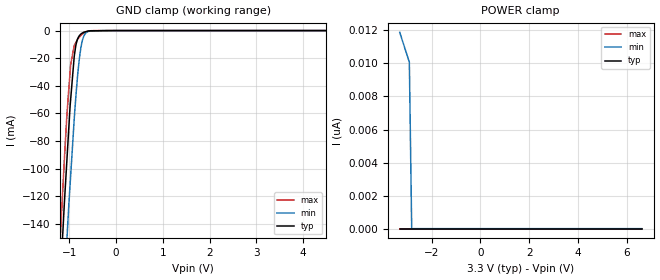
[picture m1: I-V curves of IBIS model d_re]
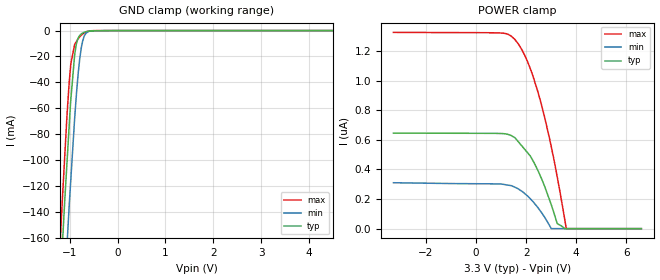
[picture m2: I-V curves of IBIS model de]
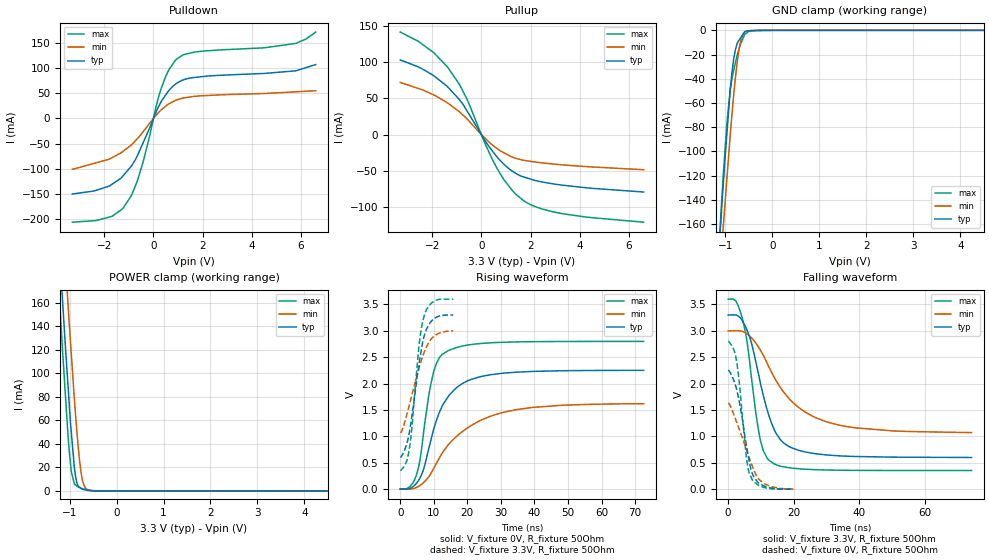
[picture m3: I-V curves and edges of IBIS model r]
|Texas Instruments Incorporated
| Robust Compact 3.3V-supply RS-485
| Marketing part#   Digital Voltage Range   Package-type   #pins
| SN65HVD75D   3V-3.6V   SOIC   8
[IBIS Ver]   3.2
[File name]   sn65hvd75.ibs
|SIMDE Ver   V3.0 - 201101 - RHL4 - Build 457
[File Rev]   1.2
[Date]   3/29/2012
[Source]
| Texas Instruments Incorporated.
| Analog-eLab Design Center, HPA
| 12500 TI Blvd
| Dallas, TX -75243
| e-mail: elab_scm_ibis@list.ti.com
[Notes]   Revision History:
| Rev 1.2: 3/29/2012
| - The VT Tables in the IBIS file are generated with
|   vfixture = Vcm(1.956-TYP, 1.731-SLOW, 2.134-FAST).
| Rev 1.1: 3/27/2012
| - IBIS file is generated with Rload = 27 Ohms &
|   Common Mode Voltage(Vcm) values calculated using the
|   setup from the datasheet.
| Rev 1.0: 3/21/2012
| - Initial version of the model
| - Model generated from simulations in TISPICE
| - Model matched to SPICE simulation
| - C_comp although listed in numerical order of value are
|   obtained from varying PVT conditions. For PVT conditions for
|   each specific value refer the buffer description under
|   respective [Model]. IBIS model user is responsible for using
|   appropriate C_comp to simulate for Signal Integrity.
|* EXCEPTION:   *
|* - For model d_re, there is leakage current in the GND   *
|*   clamp I-V Table because of the pullup on pad.   *
|* - For model de, there is leakage current in the POWER   *
|*   clamp I-V Table because of the pulldown on pad.   *
|* - For models a_b_p and a_b_n, there is leakage current in the   *
|*   POWER clamp I-V Table because of the pulldown resistors and   *
|*   the resistor network connected to pad and in the GND clamp I-V *
|*   table because of the resistor network connected to pad.   *
|* - For a_b_p and a_b_n models, pullup non-montonicity reflects   *
|*   true buffer behavior.   *
[Disclaimer]
| This model is designed as an aid for customers of Texas Instruments.
| TI and its licensors and suppliers make no warranties, either expressed
| or implied, with respect to this  model, including the warranties of
| merchantability or fitness for a particular purpose. The model is
| provided solely on an "as is" basis. The entire risk as to its quality
| and performance is with the customer.
[Copyright]
(C) Copyright 2011 Texas Instruments Incorporated.All rights reserved.
|   SN65HVD75D
[Component]   SN65HVD75D
[Manufacturer]   TI
[Package]   |8 SOIC   -  D package
|   typ   min   max
R_pkg   0.05962   0.05594   0.06721
L_pkg   2.46828nH   2.21379nH   2.98434nH
C_pkg   0.38513pF   0.35622pF   0.44246pF
[Pin]  signal_name   model_name   R_pin   L_pin   C_pin
1   R   r   0.06721   2.98434nH  0.44246pF
2   _RE   d_re   0.05732   2.24625nH  0.35866pF
3   DE   de   0.05594   2.21379nH  0.35622pF
4   D   d_re   0.06108   2.82596nH  0.43337pF
5   GND   gnd   0.02940   2.20778nH  0.47000pF
6   A   a_b_p   0.05797   2.26926nH  0.35995pF
7   B   a_b_n   0.05821   2.27008nH  0.36013pF
8   VCC   power   0.03012   2.24722nH  0.47300pF
[Diff_pin]   inv_pin   vdiff   tdelay_typ   tdelay_min   tdelay_max
6   7   0.2V   NA   NA   NA
| Models and submodels in the file (5): d_re (Input), de (Input), r (3-state), a_b_p (I/O), a_b_n (I/O)
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|   d_re Model
[Model]   d_re
Model_type   Input
Vinl = 0.8
Vinh = 2
|   typ   min   max
|   (nom PVT)   (fast PVT)   (slow PVT)
C_comp   7.616e-13   7.309e-13   8.232e-13
| Where nom  PVT is Nominal Process, 3.3V, 27C
|   Fast PVT is Strong Process,  3.6V, -40C
|   Slow PVT is Weak Process,   3V, 125C
[Voltage Range]   3.3   3   3.6
|Ambient Temperature   25   125   -40
|Junction Temperature
[Temperature Range]   27   125   -40
[Power Clamp Reference]   3.3   3   3.6
[GND Clamp Reference]   0   0   0
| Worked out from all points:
|   GND clamp passes 1 mA (typ) near -0.67 V on its own axis
[GND Clamp]
|   Voltage   I(typ)   I(min)   I(max)
-3.3V     -1.705A    -1.7A      -1.738A
-1.195V   -180.4mA   -237.2mA   -148.9mA
-1.158V   -156.2mA   -213.2mA   -124.7mA
-1.112V   -126.4mA   -185.5mA   -94.94mA
-1.055V   -93.52mA   -150.9mA   -60.84mA
-975.6mV  -50.1mA    -105.4mA   -24.74mA
-897.6mV  -18.42mA   -63.54mA   -10.82mA
-858mV    -9.846mA   -45.32mA   -8.298mA
-792mV    -3.842mA   -21.25mA   -4.834mA
-693mV    -1.196mA   -3.902mA   -1.803mA
-285mV    -93.15uA   -1.769uA   -4.655uA
6.6V      0A         0A         0A
[POWER Clamp]
|   Voltage   I(typ)   I(min)   I(max)
-3.3V     0A         11.88nA    0A
-3.298V   0A         11.87nA    0A
-3V       0A         10.5nA     0A
-2.907V   0A         10.07nA    0A
-2.811V   0A         0A         0A
6.6V      0A         0A         0A
|   de Model
[Model]   de
Model_type   Input
Vinl = 0.8
Vinh = 2
|   typ   min   max
|   (nom PVT)   (fast PVT)   (slow PVT)
C_comp   7.616e-13   7.309e-13   8.232e-13
| Where nom  PVT is Nominal Process, 3.3V, 27C
|   Fast PVT is Strong Process,  3.6V, -40C
|   Slow PVT is Weak Process,   3V, 125C
[Voltage Range]   3.3   3   3.6
|Ambient Temperature   25   125   -40
|Junction Temperature
[Temperature Range]   27   125   -40
[Power Clamp Reference]   3.3   3   3.6
[GND Clamp Reference]   0   0   0
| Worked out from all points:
|   GND clamp passes 1 mA (typ) near -0.67 V on its own axis
[GND Clamp]
|   Voltage   I(typ)   I(min)   I(max)
-3.3V     -1.872A    -1.872A    -1.901A
-1.192V   -192.8mA   -257.5mA   -157.9mA
-1.152V   -164.4mA   -228.9mA   -129.2mA
-1.105V   -132.4mA   -198mA     -97.99mA
-1.055V   -100.7mA   -164.3mA   -64.15mA
-975.6mV  -52.85mA   -114.1mA   -25.21mA
-897.6mV  -18.95mA   -68.11mA   -10.83mA
-858mV    -9.962mA   -48.2mA    -8.3mA
-792mV    -3.844mA   -22.19mA   -4.834mA
-693mV    -1.196mA   -3.944mA   -1.803mA
-285mV    -92.82uA   -1.603uA   -3.947uA
6.6V      0A         0A         0A
[POWER Clamp]
|   Voltage   I(typ)   I(min)   I(max)
-3.3V     645nA      310.1nA    1.325uA
939.6mV   642.6nA    301.8nA    1.322uA
1.422V    626.9nA    289.4nA    1.298uA
1.685V    587.5nA    268.5nA    1.248uA
1.948V    534.5nA    236.2nA    1.169uA
2.168V    490.1nA    201.3nA    1.079uA
2.473V    391.4nA    141.5nA    921.2nA
2.736V    286.6nA    77.39nA    753.7nA
3.003V    161.7nA    0A         553nA
3.241V    34.27nA    0A         349.4nA
3.604V    0A         0A         0A
6.6V      0A         0A         0A
|   r Model
[Model]   r
Model_type   3-state
Polarity   Non-Inverting
Vmeas = 1.65
Vref = 1.65
Cref = 2pF
Rref = 50
|   typ   min   max
|   (nom PVT)   (fast PVT)   (slow PVT)
C_comp   2.780e-12   2.415e-12   2.953e-12
|ON state : BUFFER OUTPUT TURNED HIGH
|C_comp   2.780e-12   2.415e-12   2.953e-12
|OFF state: BUFFER IN HIGH IMPEDANCE
|C_comp   2.507e-12   2.233e-12   2.622e-12
| Where nom  PVT is Nominal Process, 3.3V, 27C
|   Fast PVT is Strong Process,  3.6V, -40C
|   Slow PVT is Weak Process,   3V, 125C
[Voltage Range]   3.3   3   3.6
|Ambient Temperature   25   125   -40
|Junction Temperature
[Temperature Range]   27   125   -40
[Pullup Reference]   3.3   3   3.6
[Pulldown Reference]   0   0   0
[Power Clamp Reference]   3.3   3   3.6
[GND Clamp Reference]   0   0   0
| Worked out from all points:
|   slope of the pulldown table from 0 to 0.495 V, typ, clamps not added: 10.7 ohm
|   slope of the pullup table from 0 to 0.495 V, typ, clamps not added: 20.1 ohm
|   GND clamp passes 1 mA (typ) near -0.58 V on its own axis
|   POWER clamp passes 1 mA (typ) near -0.68 V on its own axis
|   falling waveform, V_fixture 3.3V, R_fixture 50Ohm: 20-80 % time 6.84ns typ, 13.6ns min, 4.27ns max; typ from 3.3 V to 0.6 V
|   rising waveform, V_fixture 0V, R_fixture 50Ohm: 20-80 % time 7.58ns typ, 14.3ns min, 4.13ns max; typ from 0 V to 2.25 V
|   rising waveform, V_fixture 3.3V, R_fixture 50Ohm: 20-80 % time 3.71ns typ, 5.13ns min, 2.82ns max; typ from 0.601 V to 3.3 V
|   falling waveform, V_fixture 0V, R_fixture 50Ohm: 20-80 % time 3.74ns typ, 5.69ns min, 2.65ns max; typ from 2.25 V to 0 V
[Pulldown]
|   Voltage   I(typ)   I(min)   I(max)
-3.3V     -149.9mA   -101.1mA   -205.7mA
-1.685V   -130.5mA   -77.82mA   -194mA
-1.249V   -114.5mA   -65.67mA   -178.9mA
-896.4mV  -94.5mA    -52.63mA   -153mA
-673.2mV  -76.17mA   -41.18mA   -126.5mA
-428.4mV  -49.17mA   -26.94mA   -87.39mA
306mV     32.4mA     16.57mA    58.12mA
633.6mV   55.83mA    28.96mA    96.76mA
939.6mV   69.38mA    36.44mA    117.2mA
1.706V    81.24mA    43.83mA    131.5mA
5.771V    94.09mA    52.55mA    148.3mA
6.6V      106.6mA    54.73mA    170.9mA
[GND Clamp]
|   Voltage   I(typ)   I(min)   I(max)
-3.3V     -1.695A    -1.623A    -1.774A
-1.168V   -200.9mA   -231.6mA   -200.3mA
-1.069V   -140.8mA   -175.9mA   -134.8mA
-1.044V   -126.3mA   -161.7mA   -119.2mA
-968.4mV  -85.6mA    -123mA     -76.83mA
-896.4mV  -49.17mA   -86.21mA   -48.82mA
-825mV    -24.16mA   -54.22mA   -33.37mA
-714mV    -8.511mA   -16.89mA   -15.83mA
-645mV    -4.403mA   -5.377mA   -8.386mA
-590.7mV  -1.17mA    -1.748mA   -3.672mA
-439.2mV  -342.9uA   -399uA     -96.91uA
6.6V      0A         0A         0A
[Pullup]
|   Voltage   I(typ)   I(min)   I(max)
-3.3V     103.4mA    72.24mA    141.8mA
-2.56V    93.6mA     63.82mA    129mA
-1.926V   81.19mA    54.79mA    113mA
-1.375V   66.16mA    43.89mA    93.4mA
-896.4mV  48.62mA    31.69mA    69.68mA
-572.4mV  32.23mA    21.44mA    48.14mA
172.8mV   -9.472mA   -5.689mA   -14.19mA
633.6mV   -30.76mA   -19.2mA    -46.34mA
1.246V    -50.27mA   -30.87mA   -76.8mA
1.706V    -58.35mA   -35.31mA   -91.08mA
3.287V    -69.84mA   -41.73mA   -109.2mA
6.6V      -79.34mA   -48.49mA   -121mA
[POWER Clamp]
|   Voltage   I(typ)   I(min)   I(max)
-3.3V     1.726A     1.768A     1.712A
-1.277V   248.4mA    321.2mA    207.4mA
-1.155V   166.1mA    237.6mA    123.2mA
-1.037V   92.04mA    161.7mA    49.65mA
-964.8mV  50.85mA    117.8mA    16.73mA
-897.6mV  19.75mA    78.19mA    5.955mA
-867.9mV  11.2mA     62.54mA    4.838mA
-816mV    4.299mA    37.54mA    3.5mA
-745.8mV  1.73mA     13.5mA     2.285mA
-657mV    822.1uA    2.18mA     1.302mA
-486mV    181.5uA    98.8uA     38.01uA
6.6V      0A         0A         0A
[Ramp]
R_load = 50
|   typ   min   max
dV/dt_r   1.35124/7.57455e-09   0.974782/1.44691e-08   1.67977/4.13078e-09
dV/dt_f   1.6192/6.82107e-09   1.15786/1.36049e-08   1.9482/4.2637e-09
[Falling Waveform]
V_fixture = 3.3V
V_fixture_min = 3V
V_fixture_max = 3.6V
R_fixture = 50Ohm
|   Time   V(typ)   V(min)   V(max)
0s        3.3V       3V         3.6V
2.275ns   3.301V     3.002V     3.571V
4.225ns   3.204V     2.992V     3.258V
5.775ns   3.013V     2.943V     2.79V
7ns       2.794V     2.876V     2.17V
9.8ns     2.023V     2.64V      937.6mV
13.27ns   1.245V     2.212V     512.1mV
18.48ns   811mV      1.724V     407.3mV
30.2ns    647.2mV    1.273V     362.7mV
74.33ns   600.3mV    1.073V     352.9mV
[Rising Waveform]
V_fixture = 0V
V_fixture_min = 0V
V_fixture_max = 0V
R_fixture = 50Ohm
|   Time   V(typ)   V(min)   V(max)
0s        613pV      31.56nV    241.3pV
4.65ns    95.64mV    25.6mV     238.5mV
5.825ns   206mV      65.75mV    532.6mV
6.875ns   359.9mV    118.2mV    1.03V
9.825ns   1.103V     374.4mV    2.192V
11.77ns   1.473V     602.2mV    2.502V
14.35ns   1.76V      841.6mV    2.626V
20.42ns   2.061V     1.177V     2.734V
31.13ns   2.199V     1.461V     2.784V
72.52ns   2.251V     1.618V     2.8V
[Rising Waveform]
V_fixture = 3.3V
V_fixture_min = 3V
V_fixture_max = 3.6V
R_fixture = 50Ohm
|   Time   V(typ)   V(min)   V(max)
0s        601.3mV    1.07V      353mV
1.775ns   822.7mV    1.37V      506.4mV
2.8ns     1.103V     1.619V     800mV
3.55ns    1.422V     1.803V     1.213V
5.625ns   2.38V      2.292V     2.749V
6.325ns   2.654V     2.449V     3.062V
7.3ns     2.94V      2.619V     3.318V
8.9ns     3.154V     2.82V      3.499V
10.43ns   3.244V     2.91V      3.576V
15.78ns   3.299V     2.999V     3.6V
[Falling Waveform]
V_fixture = 0V
V_fixture_min = 0V
V_fixture_max = 0V
R_fixture = 50Ohm
|   Time   V(typ)   V(min)   V(max)
0s        2.252V     1.625V     2.8V
1.675ns   2.068V     1.423V     2.65V
2.6ns     1.886V     1.267V     2.414V
3.525ns   1.614V     1.111V     1.94V
5.6ns     821.8mV    745.8mV    576.5mV
6.675ns   445.5mV    549.1mV    263.2mV
8ns       217.4mV    338.8mV    127.5mV
9.175ns   124.8mV    206.4mV    78.67mV
11.15ns   56.18mV    101.8mV    29.28mV
19.88ns   237.1uV    1.192mV    115.1uV
